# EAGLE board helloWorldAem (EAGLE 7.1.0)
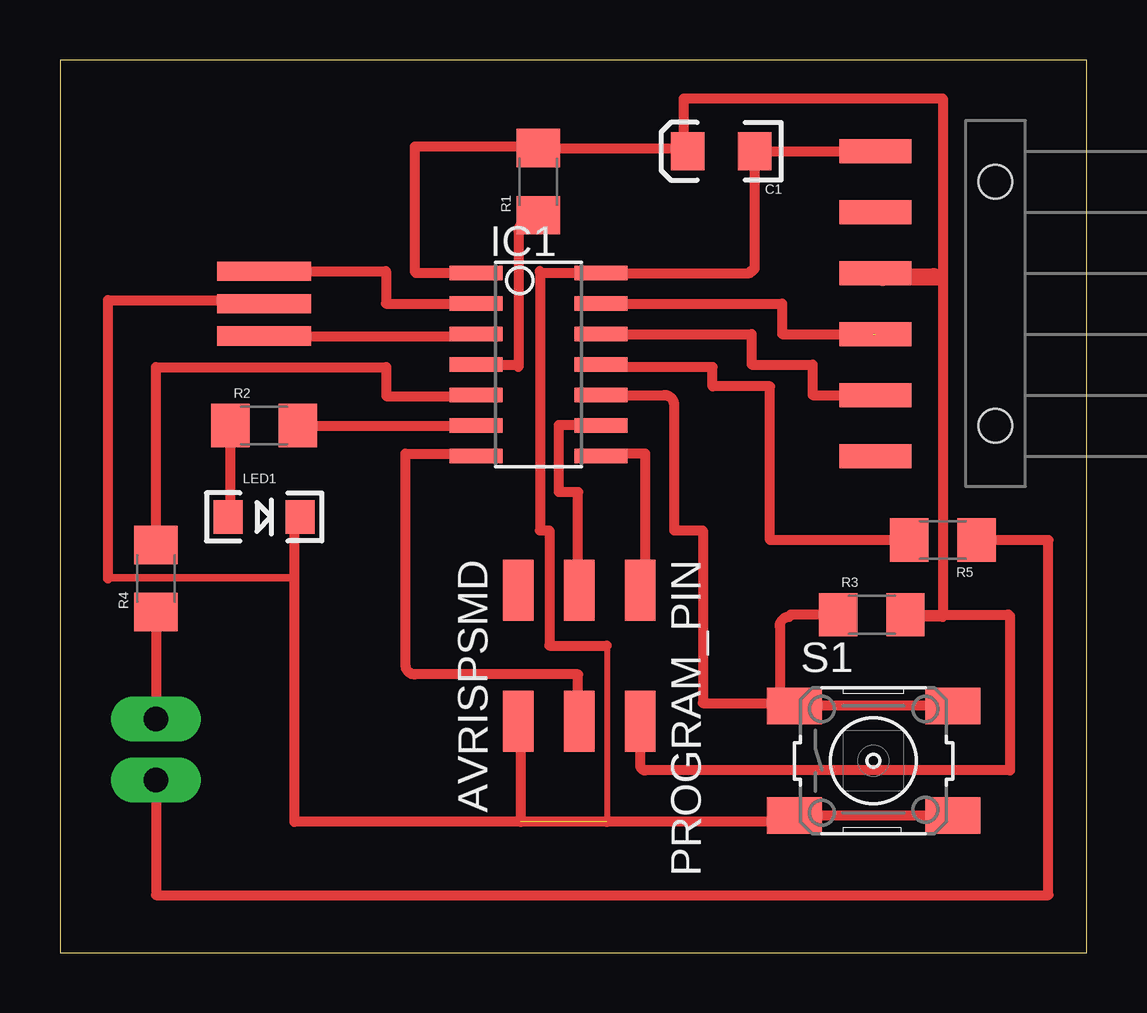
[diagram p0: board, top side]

Size 42.8 x 37.2 mm. Coordinates in mm from the lower left corner, seen from the top.
Outline: 0,0 42.8,0 42.8,37.2 0,37.2 0,0
Copper layers (1*16): Top 0.035mm / dielectric 1.5mm / Bottom 0.035mm
Design rules "default *": minimum track width 15mil, minimum drill 24mil, track to track 15mil, track to pad 15mil, pad to pad 15mil, via to via 15mil, smd to smd 15mil, copper to edge 40mil, drill to drill 8mil, minimum pad ring 10mil, minimum via ring 8mil, stop-mask expansion 4mil, vias tented up to drill 0mil, thermal gap 10mil

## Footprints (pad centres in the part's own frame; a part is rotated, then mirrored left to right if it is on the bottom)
EIA3216 = smd 1.4 x 1.6: A 1.4,0; C -1.4,0
SOIC14 = smd 0.61 x 2.21: 1 -3.81,-2.603; 2 -2.54,-2.603; 3 -1.27,-2.603; 4 0,-2.603; 5 1.27,-2.603; 6 2.54,-2.603; 7 3.81,-2.603; 8 3.81,2.603; 9 2.54,2.603; 10 1.27,2.603; 11 0,2.603; 12 -1.27,2.603; 13 -2.54,2.603; 14 -3.81,2.603
1X06-SMD = smd 1 x 3: 1 -6.35,5; 2 -3.81,5; 3 -1.27,5; 4 1.27,5; 5 3.81,5; 6 6.35,5 | hole 1.4: -5.08,0; 5.08,0
1X02_LONGPADS = drill 1.016 pad 1.88 long: 1 0,0; 2 2.54,0
LED-1206 = smd 1.2 x 1.4: A -1.5,0; C 1.5,0
2X03SMD = smd 2.54 x 1.27: 1 -2.54,2.54; 2 2.92,2.54; 3 -2.54,0; 4 2.92,0; 5 -2.54,-2.54; 6 2.92,-2.54
1206 = smd 1.6 x 1.8: 1 -1.4,0; 2 1.4,0
EFOBM = smd 0.8 x 3.9: 1 -1.35,0; 2 0,0; 3 1.35,0
6MM_SWITCH = smd 2.286 x 1.524: 1 -3.302,2.286; 2 3.302,2.286; 3 -3.302,-2.286; 4 3.302,-2.286

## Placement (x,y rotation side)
C1  1uF  [EIA3216]  27.56,33.4 180 top
IC1  ATTINY44-SSU  [SOIC14]  19.94,24.51 270 top
INTERFACE  [1X06-SMD]  38.99,27.05 90 top
JP2  [1X02_LONGPADS]  4,7.2 90 top
LED1  [LED-1206]  8.51,18.16 0 top
PROGRAM_PIN  AVRISPSMD  [2X03SMD]  21.65,12.57 270 top
R1  10k  [1206]  19.94,32.13 90 top
R2  100  [1206]  8.51,21.97 0 top
R3  10k  [1206]  33.84,14.09 0 top
R4  0  [1206]  4,15.6 90 top
R5  0  [1206]  36.8,17.2 180 top
RESONATOR  RESONATOR  [EFOBM]  8.51,27.05 270 top
S1  [6MM_SWITCH]  33.91,8 0 top

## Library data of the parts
C1 INTERFACE JP2 LED1 R1-R5 = 01_SparkFun
IC1 PROGRAM_PIN RESONATOR S1 = fab

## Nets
BTN: IC1.10 R3.1 S1.1 S1.2
CTS: INTERFACE.5
GND: C1.C IC1.14 INTERFACE.6 LED1.C PROGRAM_PIN.6 RESONATOR.2 S1.3 S1.4
LED: IC1.6 R2.2
MISO: IC1.8
MOSI: IC1.7 PROGRAM_PIN.4
N$1: JP2.2 R4.1
N$2: IC1.3 RESONATOR.3
N$3: IC1.2 RESONATOR.1
N$4: LED1.A R2.1
N$5: JP2.1 R5.1
PIN5: IC1.5 R4.2
PIN11: IC1.11 R5.2
RST: IC1.4 R1.1
RTS: INTERFACE.1
RX: IC1.12 INTERFACE.2
SCK: IC1.9
TX: IC1.13 INTERFACE.3
VCC: C1.A IC1.1 INTERFACE.4 PROGRAM_PIN.2 R1.2 R3.2

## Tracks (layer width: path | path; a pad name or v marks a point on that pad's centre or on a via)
BTN
  Top 0.406: S1.2 31.2,10.29 | 31.2,10.29 S1.1 | IC1.10 25.19,23.24 arc-90 25.6,22.83 25.6,17.6 26.8,17.6 26.8,10.4 30,10.4 | 30,10.4 31.09,10.4 arc-90 31.2,10.29 | R3.1 30.49,14.09 arc90 30.4,14 arc90 30,13.6 30,10.4
GND  (2 unrouted)
  Top 0.254: 22.8,12.8 22.8,5.46
  Top 0.305: 2.02,15.62 9.76,15.62 arc-90 9.78,15.6
  Top 0.406: S1.4 31.37,5.71 | 31.37,5.71 S1.3 | 31.37,5.71 31.37,5.46 22.8,5.46 19.2,5.46 | 19.2,5.46 9.78,5.46 9.78,15.6 9.78,17.93 arc-90 LED1.C | INTERFACE.6 C1.C 28.96,28.56 arc-90 28.8,28.4 arc-90 28.72,28.32 IC1.14 20.08,28.32 arc-90 20,28.4 20,17.6 20.4,17.6 20.4,12.8 22.8,12.8 | PROGRAM_PIN.6 arc-90 19.2,9.56 19.2,5.46 | 2.02,15.62 arc90 2,15.6 2,27.2 8.36,27.2 arc-90 RESONATOR.2
LED
  Top 0.406: R2.2 IC1.6
MISO
  Top 0.406: 24.4,15.32 24.4,20.8 22.64,20.8 arc90 IC1.8
MOSI
  Top 0.406: PROGRAM_PIN.4 arc-90 21.6,9.7 21.6,11.6 14.8,11.6 arc-90 14.4,12 14.4,20.8 17.24,20.8 arc-90 IC1.7
N$1
  Top 0.406: R4.1 JP2.2
N$2
  Top 0.406: 17.34,25.7 IC1.3 17.26,25.7 RESONATOR.3
N$3
  Top 0.406: RESONATOR.1 13.59,28.4 13.59,27.05 IC1.2
N$4
  Top 0.406: LED1.A 7.11,18.16 R2.1
N$5
  Top 0.406: JP2.1 4,2.4 41.2,2.4 41.2,17.2 R5.1
PIN5
  Top 0.406: R4.2 4,24.4 13.6,24.4 13.6,23.2 17.3,23.2 arc90 IC1.5
PIN11
  Top 0.406: R5.2 29.6,17.2 29.6,23.6 27.2,23.6 27.2,24.4 22.65,24.4 arc-90 IC1.11
RST
  Top 0.406: R1.1 19.75,30.73 arc90 19.43,30.41 arc90 19.11,30.09 19.11,24.4 arc90 19,24.51 IC1.4
RX
  Top 0.406: IC1.12 28.83,25.78 28.83,24.51 31.37,24.51 31.37,23.24 INTERFACE.2
SCK
  Top 0.406: 21.6,15.16 21.6,19.2 20.8,19.2 20.8,22 22.51,22 arc-90 IC1.9
TX  (1 unrouted)
  Top 0.406: IC1.13 30.1,27.05 30.1,25.78 33.91,25.78
VCC
  Top 0.406: IC1.1 14.88,28.32 arc-90 14.8,28.4 14.8,33.6 19.87,33.6 arc-90 R1.2 26.03,33.53 arc-90 C1.A arc-90 26,33.56 26,35.6 36.8,35.6 36.8,28 34.31,28 arc-90 INTERFACE.4 36.39,28.32 arc-90 36.8,27.91 36.8,14 35.33,14 arc-90 R3.2 39.51,14.09 arc-90 39.6,14 39.6,7.6 24.4,7.6 arc-90 24.19,7.81 PROGRAM_PIN.2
